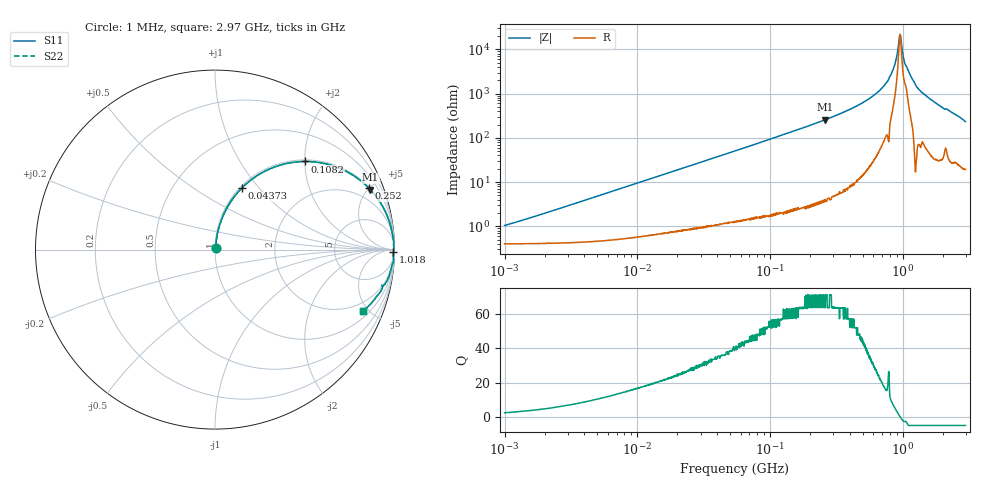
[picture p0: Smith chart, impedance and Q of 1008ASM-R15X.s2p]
!s-Parameter Generated by FASTRON Sdn. Bhd.
!FASTRON P/N : 1008ASM-R15X
!Keysight Technologies: E4991B_MY54100416_A.01.15
!Date: Mon Nov 20 16:11:49 2023
!Version  :Rev00  Wed Nov 22 15:12:57 2023
!Data & Calibration Information:
!Freq  S11  S21  S12  S22
!PortZ  Port1:50+j0  Port2:50+j0
!When reading reference impedance value at option line is always used.
! Remarks : This data is being provided solely for informational purposes.
# Hz S dB R 50
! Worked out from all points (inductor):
!   1599 points, 1 MHz to 2.97 GHz, reference 50 ohm
!   read as one part in series: L = 153 nH near 1.253 MHz
!   highest Q = 71.2 at 261 MHz (marker M1), where L = 157 nH
!   self-resonance near 953.8 MHz
!   S11 on the Smith chart (normalised r, x): 1 MHz: 1.01, +0.02; 43.73 MHz: 1.02, +0.81; 108.2 MHz: 1.04, +2.01; 252 MHz: 1.07, +4.94; 1.018 GHz: open; 2.97 GHz: 1.39, -4.63
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1000000  -39.70 66.9  -0.04 -0.6  -0.04 -0.6  -39.70 66.9
3804036  -28.70 81.1  -0.04 -2.1  -0.04 -2.1  -28.70 81.1
1.439846e7  -17.50 79.5  -0.14 -7.7  -0.14 -7.7  -17.50 79.5
4.37287e7  -8.56 66.5  -0.75 -21.9  -0.75 -21.9  -8.56 66.5
5.477226e7  -6.96 61.9  -1.09 -26.7  -1.09 -26.7  -6.96 61.9
1.081723e8  -3.06 44.3  -3.12 -44.7  -3.12 -44.7  -3.06 44.3
2.073156e8  -1.03 26.5  -7.01 -62.6  -7.01 -62.6  -1.03 26.5
2.519921e8  -0.70 21.9  -8.57 -67.3  -8.57 -67.3  -0.70 21.9
2.609752e8  -0.65 21.1  -8.87 -68.0  -8.87 -68.0  -0.65 21.1
5.418594e8  -0.11 7.8  -17.30 -80.6  -17.30 -80.6  -0.11 7.8
6.821091e8  -0.06 4.6  -22.00 -82.8  -22.00 -82.8  -0.06 4.6
7.846996e8  -0.02 2.6  -26.70 -85.2  -26.70 -85.2  -0.02 2.6
8.672962e8  -0.04 1.3  -32.70 -78.6  -32.70 -78.6  -0.04 1.3
9.302341e8  -0.04 0.4  -42.20 -56.3  -42.20 -56.3  -0.04 0.4
9.490412e8  -0.04 0.1  -46.40 -21.7  -46.40 -21.7  -0.04 0.1
9.730857e8  -0.04 -0.2  -44.10 41.1  -44.10 41.1  -0.04 -0.2
1.017911e9  -0.05 -0.9  -35.90 67.8  -35.90 67.8  -0.05 -0.9
1.054198e9  -0.07 -1.2  -32.90 68.3  -32.90 68.3  -0.07 -1.2
1.136371e9  -0.05 -2.1  -28.60 80.3  -28.60 80.3  -0.05 -2.1
1.353887e9  -0.07 -4.8  -21.40 82.0  -21.40 82.0  -0.07 -4.8
1.941122e9  -0.26 -10.9  -14.40 75.6  -14.40 75.6  -0.26 -10.9
2.970126e9  -1.00 -22.5  -8.30 62.7  -8.30 62.7  -1.00 -22.5
